{attribute 'call_after_init'}
{attribute 'reflection'} 
FUNCTION_BLOCK FB_Log IMPLEMENTS I_SendLog

VAR
	{attribute 'hide'}
	_aLogBaseExt 				: ARRAY[-1..SIZEOF(TwinCAT_SystemInfoVarList._TaskInfo)/SIZEOF(PlcTaskSystemInfo)] OF FB_LogBaseExt;
	{attribute 'hide'}
	_aInternalMsg				: ARRAY[-1..SIZEOF(TwinCAT_SystemInfoVarList._TaskInfo)/SIZEOF(PlcTaskSystemInfo)] OF STRING(100);
	{attribute 'hide'}
	_aLogSeverity				: ARRAY[-1..SIZEOF(TwinCAT_SystemInfoVarList._TaskInfo)/SIZEOF(PlcTaskSystemInfo)] OF E_Severity;
	
	{attribute 'hide'}
	{attribute 'instance-path'} 
    {attribute 'noinit'} 
    _InstancePath 					: STRING; 						// contains instance path 	


	{attribute 'hide'}
	_bUseExternalName				: BOOL;
	_InstanceName 					: STRING(25);


END_VAR

METHOD Protected _GetLogConditionFullfilled : BOOL
VAR_INPUT
	eSeverity	: E_Severity;
END_VAR
 // Each Tasklogger is configured identically, therefore it is sufficient to check the first.
_GetLogConditionFullfilled := _aLogBaseExt[1].GetLogConditionFullfilled(eSeverity);
END_METHOD

{attribute 'call_after_init'}
METHOD protected _Init

VAR_INST
	i					:	UINT;
	_sShortenedPath		:	T_MAXSTRING;
	_nPosInString		:	INT := 0;
END_VAR
// Get Instance Path
IF NOT _bUseExternalName THEN
	_sShortenedPath := _InstancePath;
	
	WHILE(FIND(_sShortenedPath, '.') > 0) DO
		_nPosInString := FIND(_sShortenedPath, '.');
		_sShortenedPath := DELETE(_sShortenedPath, _nPosInString+1, 0);	
	END_WHILE

	_InstanceName := _sShortenedPath;
	Name := _sShortenedPath;
END_IF
END_METHOD

METHOD AddString : I_SendLog
VAR_INPUT
	sString	: STRING(50);
END_VAR
IF _aLogSeverity[Tc2_System.GETCURTASKINDEXEX()] <> E_Severity.off THEN
	_aInternalMsg[Tc2_System.GETCURTASKINDEXEX()] := Concat(_aInternalMsg[Tc2_System.GETCURTASKINDEXEX()],sString);
END_IF
AddString := THIS^;
END_METHOD

{attribute 'hasanytype'}
METHOD AddVar : I_SendLog

VAR_INPUT
	{attribute 'anytypeclass' := 'ANY'}
	anyVar	: __SYSTEM.AnyType;
END_VAR
IF _aLogSeverity[Tc2_System.GETCURTASKINDEXEX()] <> E_Severity.off THEN
	_aInternalMsg[Tc2_System.GETCURTASKINDEXEX()] := Concat(_aInternalMsg[Tc2_System.GETCURTASKINDEXEX()],TO_STRING(anyVar.pValue^));
END_IF
AddVar := THIS^;
END_METHOD

METHOD Debug : I_SendLog
VAR_INPUT
	sMsg	: STRING(25);
END_VAR
IF _GetLogConditionFullfilled(eSeverity := E_Severity.debug) THEN
	_aLogSeverity[Tc2_System.GETCURTASKINDEXEX()] := E_Severity.debug;
	_aInternalMsg[Tc2_System.GETCURTASKINDEXEX()] := sMsg;
ELSE
	_aLogSeverity[Tc2_System.GETCURTASKINDEXEX()] := E_severity.off;
END_IF

Debug := THIS^;
END_METHOD

METHOD Error : I_SendLog
VAR_INPUT
	sMsg : STRING(25);
END_VAR
IF _GetLogConditionFullfilled(eSeverity := E_Severity.error) THEN
	_aLogSeverity[Tc2_System.GETCURTASKINDEXEX()] := E_Severity.error;
	_aInternalMsg[Tc2_System.GETCURTASKINDEXEX()] := sMsg;
ELSE
	_aLogSeverity[Tc2_System.GETCURTASKINDEXEX()] := E_severity.off;
END_IF

Error := THIS^;
END_METHOD

METHOD Fatal : I_SendLog
VAR_INPUT
	sMsg	: STRING;
END_VAR
IF _GetLogConditionFullfilled(eSeverity := E_Severity.fatal) THEN
	_aLogSeverity[Tc2_System.GETCURTASKINDEXEX()] := E_Severity.fatal;
	_aInternalMsg[Tc2_System.GETCURTASKINDEXEX()] := sMsg;
ELSE
	_aLogSeverity[Tc2_System.GETCURTASKINDEXEX()] := E_severity.off;
END_IF

Fatal := THIS^;
END_METHOD

METHOD Info : I_SendLog
VAR_INPUT
	sMsg	: STRING;
END_VAR
IF _GetLogConditionFullfilled(eSeverity := E_Severity.info) THEN
	_aLogSeverity[Tc2_System.GETCURTASKINDEXEX()] := E_Severity.info;
	_aInternalMsg[Tc2_System.GETCURTASKINDEXEX()] := sMsg;
ELSE
	_aLogSeverity[Tc2_System.GETCURTASKINDEXEX()] := E_severity.off;
END_IF

Info := THIS^;
END_METHOD

PROPERTY PUBLIC LogCollector : I_PushLog
SET
VAR
	n : DINT;
END_VAR
FOR n := -1 TO SIZEOF(TwinCAT_SystemInfoVarList._TaskInfo)/SIZEOF(PlcTaskSystemInfo) DO
	_aLogBaseExt[n].LogCollector := LogCollector;
END_FOR
END_SET
END_PROPERTY

PROPERTY Public MinSeverity : E_Severity
SET
VAR
	n : DINT;
END_VAR
FOR n := -1 TO SIZEOF(TwinCAT_SystemInfoVarList._TaskInfo)/SIZEOF(PlcTaskSystemInfo) DO
	_aLogBaseExt[n].MinSeverity := MinSeverity;
END_FOR
END_SET
END_PROPERTY

PROPERTY Name : String(25)
SET
VAR
	n : DINT;
END_VAR
_bUseExternalName := TRUE;
_InstanceName := Name;
FOR n := -1 TO SIZEOF(TwinCAT_SystemInfoVarList._TaskInfo)/SIZEOF(PlcTaskSystemInfo) DO
	_aLogBaseExt[n].Name := Name;
END_FOR
END_SET
END_PROPERTY

METHOD Send : BOOL
IF _aLogSeverity[Tc2_System.GETCURTASKINDEXEX()] <> E_Severity.off THEN
	Send := _aLogBaseExt[Tc2_System.GETCURTASKINDEXEX()].SendMessage(sMsg := _aInternalMsg[Tc2_System.GETCURTASKINDEXEX()],
																	eSeverity := _aLogSeverity[Tc2_System.GETCURTASKINDEXEX()]);
ELSE
	Send := FALSE;
END_IF
END_METHOD

METHOD Trace : I_SendLog
VAR_INPUT
	sMsg	: STRING;
END_VAR
IF _GetLogConditionFullfilled(eSeverity := E_Severity.trace) THEN
	_aLogSeverity[Tc2_System.GETCURTASKINDEXEX()] := E_Severity.trace;
	_aInternalMsg[Tc2_System.GETCURTASKINDEXEX()] := sMsg;
ELSE
	_aLogSeverity[Tc2_System.GETCURTASKINDEXEX()] := E_severity.off;
END_IF

Trace := THIS^;
END_METHOD

METHOD Warn : I_SendLog
VAR_INPUT
	sMsg	: STRING;
END_VAR
IF _GetLogConditionFullfilled(eSeverity := E_Severity.warn) THEN
	_aLogSeverity[Tc2_System.GETCURTASKINDEXEX()] := E_Severity.warn;
	_aInternalMsg[Tc2_System.GETCURTASKINDEXEX()] := sMsg;
ELSE
	_aLogSeverity[Tc2_System.GETCURTASKINDEXEX()] := E_severity.off;
END_IF

Warn := THIS^;
END_METHOD

END_FUNCTION_BLOCK
